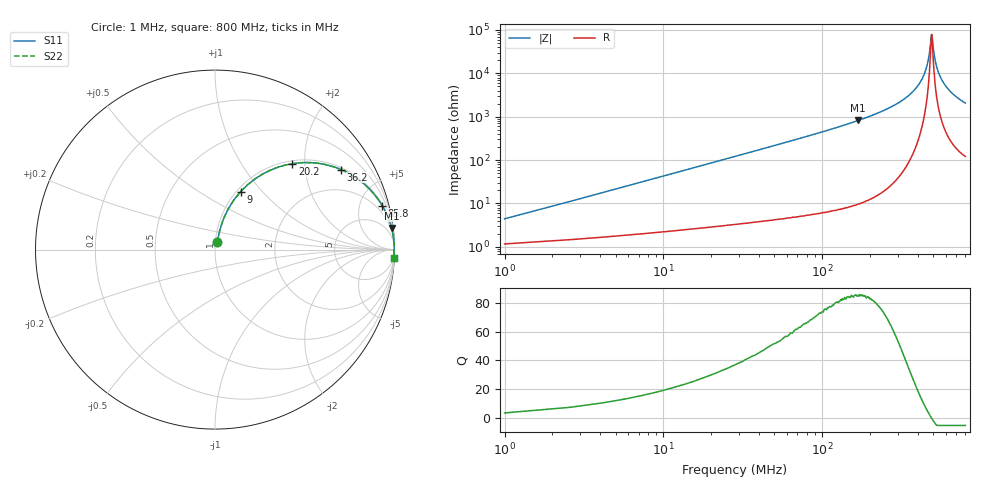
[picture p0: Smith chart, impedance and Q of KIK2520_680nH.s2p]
!version-2
!date-01.2022
!Series
# MHz S RI R 50
!Freq ReS11 ImS11 ReS21 ImS21 ReS12 ImS12 ReS22 ImS22
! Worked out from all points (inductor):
!   501 points, 1 MHz to 800 MHz, reference 50 ohm
!   read as one part in series: L = 680 nH near 4.2 MHz
!   highest Q = 85 at 169 MHz (marker M1), where L = 772 nH
!   self-resonance near 491 MHz
!   S11 on the Smith chart (normalised r, x): 1 MHz: 1.02, +0.09; 9 MHz: 1.04, +0.77; 20.2 MHz: 1.06, +1.73; 36.2 MHz: 1.07, +3.11; 85.8 MHz: 1.11, +7.56; 800 MHz: 3, -41
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1  0.0133 0.0417  0.9867 -0.0417  0.9867 -0.0417  0.0133 0.0417
5.8  0.0731 0.2256  0.9269 -0.2256  0.9269 -0.2256  0.0731 0.2256
9  0.1425 0.3229  0.8575 -0.3229  0.8575 -0.3229  0.1425 0.3229
13.8  0.2672 0.4219  0.7328 -0.4219  0.7328 -0.4219  0.2672 0.4219
20.2  0.4303 0.4788  0.5697 -0.4788  0.5697 -0.4788  0.4303 0.4788
36.2  0.7033 0.4453  0.2967 -0.4453  0.2967 -0.4453  0.7033 0.4453
55.4  0.8473 0.3506  0.1527 -0.3506  0.1527 -0.3506  0.8473 0.3506
85.8  0.9315 0.2453  0.0685 -0.2453  0.0685 -0.2453  0.9315 0.2453
135  0.9733 0.1551  0.0267 -0.1551  0.0267 -0.1551  0.9733 0.1551
169  0.984 0.1199  0.016 -0.1199  0.016 -0.1199  0.984 0.1199
268  0.9953 0.0608  0.00466 -0.0608  0.00466 -0.0608  0.9953 0.0608
401  0.9986 0.0193  0.00139 -0.0193  0.00139 -0.0193  0.9986 0.0193
435  0.9988 0.0116  0.00123 -0.0116  0.00123 -0.0116  0.9988 0.0116
459  0.9988 0.00643  0.00121 -0.00643  0.00121 -0.00643  0.9988 0.00643
475  0.9988 0.00316  0.00122 -0.00316  0.00122 -0.00316  0.9988 0.00316
487  0.9987 0.000633  0.00126 -0.000633  0.00126 -0.000633  0.9987 0.000633
491  0.9987 1.03e-05  0.00127 -1.03e-05  0.00127 -1.03e-05  0.9987 1.03e-05
511  0.9986 -0.00394  0.00136 0.00394  0.00136 0.00394  0.9986 -0.00394
534  0.9985 -0.00802  0.00149 0.00802  0.00149 0.00802  0.9985 -0.00802
583  0.9981 -0.0165  0.00191 0.0165  0.00191 0.0165  0.9981 -0.0165
667  0.9971 -0.0295  0.00292 0.0295  0.00292 0.0295  0.9971 -0.0295
800  0.9948 -0.0481  0.00517 0.0481  0.00517 0.0481  0.9948 -0.0481
